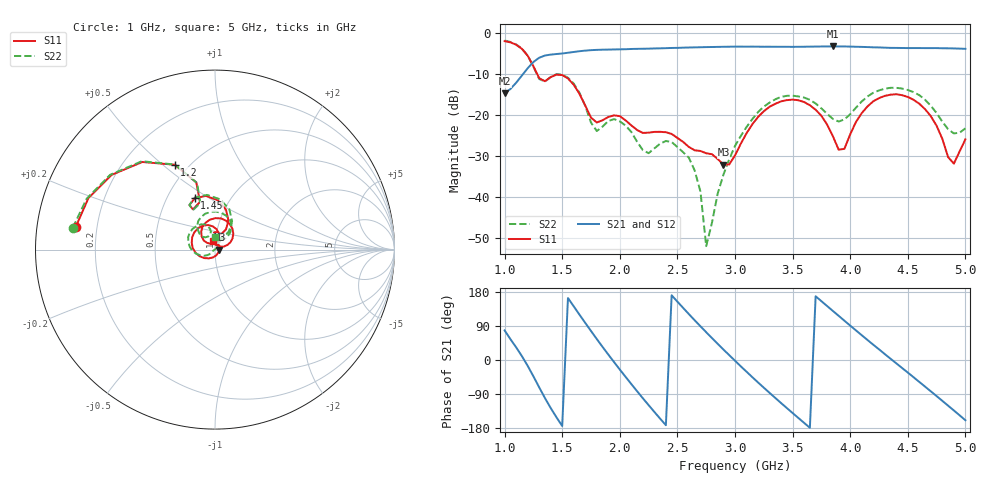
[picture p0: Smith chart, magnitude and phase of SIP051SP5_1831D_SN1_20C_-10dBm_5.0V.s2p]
# GHz  S  dB  R  50
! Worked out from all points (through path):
!   81 points, 1 GHz to 5 GHz, reference 50 ohm
!   highest |S21| = -3.37 dB at 3.85 GHz (marker M1); lowest = -14.8 dB at 1 GHz (marker M2)
!   lowest |S11| = -32.2 dB at 2.9 GHz (marker M3), VSWR 1.05, Z = 52.5 - j0.0826 ohm
!   |S11| at or under -10 dB: 1.281 GHz to end of sweep
!   |S22| runs from -52.1 to -1.9 dB; largest |S21 - S12| = 0.0024
!   S11 on the Smith chart (normalised r, x): 1 GHz: 0.12, +0.08; 1.2 GHz: 0.42, +0.55; 1.45 GHz: 0.69, +0.43; 5 GHz: 0.97, +0.09
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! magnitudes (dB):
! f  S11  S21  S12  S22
! 1 GHz  -2.1  -14.8  -14.8  -1.9
! 1.2 GHz  -5.6  -8.7  -8.7  -5.6
! 1.3 GHz  -11.1  -6.1  -6.1  -11.3
! 1.45 GHz  -10.3  -5.2  -5.2  -10.1
! 1.7 GHz  -17.8  -4.4  -4.4  -17.9
! 1.8 GHz  -21.9  -4.2  -4.2  -24.0
! 1.95 GHz  -20.2  -4.1  -4.1  -21.1
! 2.2 GHz  -24.5  -3.9  -3.9  -28.7
! 2.35 GHz  -24.2  -3.8  -3.8  -27.1
! 2.65 GHz  -28.7  -3.6  -3.6  -33.6
! 2.7 GHz  -28.9  -3.6  -3.6  -38.8
! 2.75 GHz  -29.4  -3.5  -3.5  -52.1
! 2.9 GHz  -32.2  -3.5  -3.5  -34.6
! 3 GHz  -30.0  -3.4  -3.4  -27.6
! 3.3 GHz  -18.1  -3.4  -3.4  -17.1
! 3.7 GHz  -18.8  -3.4  -3.4  -17.3
! 3.85 GHz  -25.3  -3.4  -3.4  -21.1
! 3.95 GHz  -28.3  -3.4  -3.4  -21.2
! 4.35 GHz  -15.1  -3.7  -3.7  -13.5
! 4.65 GHz  -18.7  -3.8  -3.8  -16.4
! 4.9 GHz  -32.0  -3.9  -3.9  -24.6
! 5 GHz  -26.0  -4.0  -4.0  -23.4
